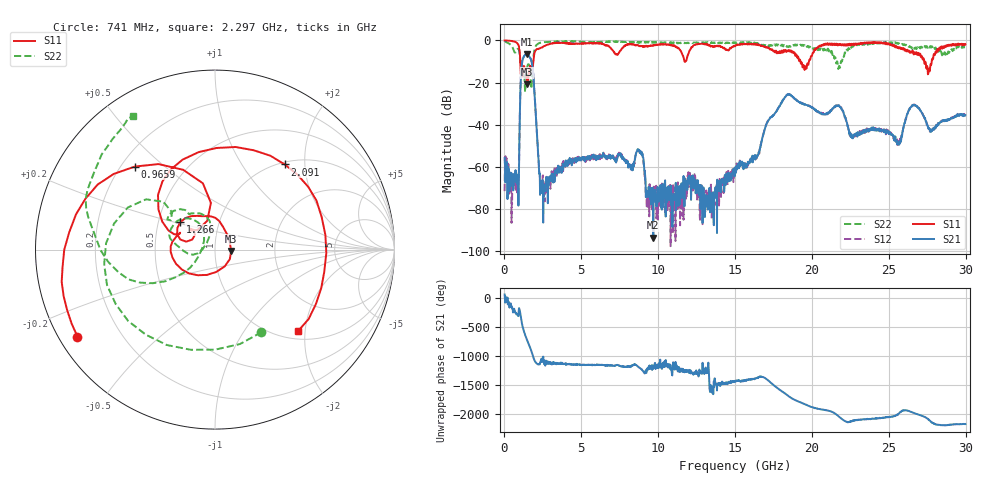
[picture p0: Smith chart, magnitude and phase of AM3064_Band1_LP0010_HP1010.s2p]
# Hz S DB R 50.0
!freq dBS11 angS11 dBS21 angS21 dBS12 angS12 dBS22 angS22
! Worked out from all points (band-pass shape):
!   1600 points, 10 MHz to 29.98 GHz, reference 50 ohm
!   highest |S21| = -6.65 dB at 1.435 GHz (marker M1); lowest = -93.6 dB at 9.682 GHz (marker M2)
!   |S21| within 3 dB of the highest: 1.169 GHz to 1.747 GHz (577.8 MHz wide, 39.6 % of centre)
!   lowest |S11| = -20.9 dB at 1.491 GHz (marker M3), VSWR 1.20, Z = 59.9 - j0.851 ohm
!   |S11| at or under -10 dB: 1.031 GHz to 1.879 GHz (847.8 MHz wide, 58.3 % of centre); 19.25 GHz to 19.8 GHz (553.5 MHz wide, 2.83 % of centre); 27.3 GHz to 27.79 GHz (487.7 MHz wide, 1.77 % of centre)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
!   |S22| runs from -24.5 to -0.3 dB; largest |S21 - S12| = 0.0055
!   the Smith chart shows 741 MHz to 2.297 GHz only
!   S11 on the Smith chart (normalised r, x): 741 MHz: 0.05, -0.29; 965.9 MHz: 0.25, +0.40; 1.266 GHz: 0.65, +0.21; 2.091 GHz: 1.04, +1.58; 2.297 GHz: 1.17, -1.84
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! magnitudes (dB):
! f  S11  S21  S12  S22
! 10 MHz  -0.1  -55.8  -71.5  -0.3
! 741 MHz  -0.9  -67.2  -70.3  -5.5
! 965.9 MHz  -3.8  -49.3  -49.0  -5.4
! 1.266 GHz  -12.2  -7.7  -7.6  -14.3
! 1.435 GHz  -17.4  -6.6  -6.6  -15.1
! 1.491 GHz  -20.9  -6.8  -6.8  -12.3
! 1.809 GHz  -13.3  -11.9  -11.8  -15.3
! 2.091 GHz  -4.3  -41.8  -41.5  -2.1
! 2.297 GHz  -3.8  -63.1  -63.8  -1.2
! 5.015 GHz  -1.4  -55.8  -56.2  -0.6
! 8.763 GHz  -2.8  -52.3  -52.9  -1.1
! 9.682 GHz  -2.4  -93.6  -70.0  -0.9
! 10 GHz  -2.0  -75.5  -73.1  -0.9
! 13.52 GHz  -2.9  -81.5  -75.7  -1.2
! 15 GHz  -2.6  -62.8  -61.4  -1.3
! 18.36 GHz  -5.2  -25.9  -26.0  -3.0
! 19.99 GHz  -7.4  -31.9  -31.8  -3.4
! 25 GHz  -1.4  -44.5  -44.2  -1.2
! 25.67 GHz  -3.8  -49.5  -47.6  -1.5
! 26.63 GHz  -6.7  -30.8  -30.4  -3.2
! 27.56 GHz  -16.0  -41.2  -41.4  -2.7
! 29.98 GHz  -1.8  -35.5  -35.5  -3.2
